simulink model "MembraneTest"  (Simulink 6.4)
settings: Solver=ode45  StartTime=0.0  StopTime=SimTime  FixedStep=1E-2  RelTol=1e-5
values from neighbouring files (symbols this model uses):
  b = S/Sm    (= 0.1)    [Constantes.m]    (also in ConstantesBck.m)
  C = 1    [Constantes.m]    (also in ConstantesBck.m)
  Cmem = 1E-6*Sm*(1-b)    (= 2.826e-08)    [Constantes.m]    (also in ConstantesBck.m = 3.14e-11; ImpedanceZtissus.m = 4e-08; Ztissus.m = 4e-08; CalculCharge.m = 1)
  Fact = 10^2    (= 100)    [Constantes.m]    (also in ConstantesBck.m)
  gk = 36    [Constantes.m]    (also in ConstantesBck.m; sim_hh.m)
  gl = 0.3    [Constantes.m]    (also in ConstantesBck.m; sim_hh.m)
  gna = 120    [Constantes.m]    (also in ConstantesBck.m; sim_hh.m)
  h0 = cdep(4)    [temps.m]    (also in Constantes.m = 0.5961; ConstantesBck.m = 0.5961)
  I0Stim = AddI    (= 0)    [WaveComp.m]    (also in WaveCompIET.m; WaveCompIETAnim.m; WaveCompIETIf.m; WaveCompIETSeul.m = Hm(i)*1E-6)
  m0 = cdep(5)    [temps.m]    (also in Constantes.m = 0.0529; ConstantesBck.m = 0.0529)
  mK = 0    [Constantes.m]    (also in ConstantesBck.m)
  mL = 0    [Constantes.m]    (also in ConstantesBck.m)
  mNa = 0    [Constantes.m]    (also in ConstantesBck.m)
  n0 = 0.3177    [Constantes.m]    (also in ConstantesBck.m)
  Rcan = 6.398E3*Sm*(1-b)    (= 180.80748)    [Constantes.m]    (also in ConstantesBck.m = 0.03454; ImpedanceZtissus.m = 44; Ztissus.m = 44)
  Sm = 3.14e-2    (= 0.0314)    [Constantes.m]    (also in ConstantesBck.m = 0.000314)
  T0Stim = i    [WaveComp.m]    (also in WaveCompIET.m; WaveCompIETAnim.m = 5; WaveCompIETIf.m; WaveCompIETSeul.m = T0Hm(i)*1E-3)
  TypeStim = 5    [WaveComp.m]    (also in WaveCompIET.m; WaveCompIETAnim.m; WaveCompIETIf.m; WaveCompIETSeul.m)
  Vk = -82    [Constantes.m]    (also in ConstantesBck.m)
  Vl = -59    [Constantes.m]    (also in ConstantesBck.m)
  Vna = 45    [Constantes.m]    (also in ConstantesBck.m)
  Vr = -70    [Constantes.m]    (also in ConstantesBck.m)
libraries: simulink x1

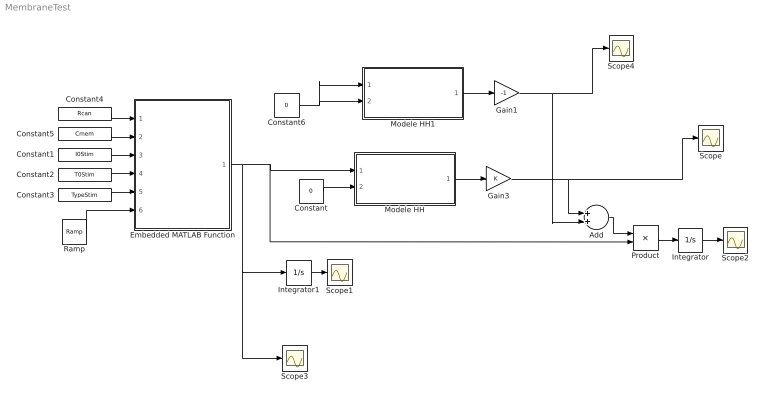
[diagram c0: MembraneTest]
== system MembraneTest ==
  Add : Sum  OutScaling=2^-10
  Constant : Constant  Value=0  OutDataType=sfix(16)  ConRadixGroup=Use specified scaling  OutScaling=2^0  SampleTime=inf  FramePeriod=inf
  Constant1 : Constant  Value=I0Stim  OutDataType=sfix(16)  ConRadixGroup=Use specified scaling  OutScaling=2^0  SampleTime=inf  FramePeriod=inf
  Constant2 : Constant  Value=T0Stim  OutDataType=sfix(16)  ConRadixGroup=Use specified scaling  OutScaling=2^0  SampleTime=inf  FramePeriod=inf
  Constant3 : Constant  Value=TypeStim  OutDataType=sfix(16)  ConRadixGroup=Use specified scaling  OutScaling=2^0  SampleTime=inf  FramePeriod=inf
  Constant4 : Constant  Value=Rcan  OutDataType=sfix(16)  ConRadixGroup=Use specified scaling  OutScaling=2^0  SampleTime=inf  FramePeriod=inf
  Constant5 : Constant  Value=Cmem  OutDataType=sfix(16)  ConRadixGroup=Use specified scaling  OutScaling=2^0  SampleTime=inf  FramePeriod=inf
  Constant6 : Constant  Value=0  OutDataType=sfix(16)  ConRadixGroup=Use specified scaling  OutScaling=2^0  SampleTime=inf  FramePeriod=inf
  Embedded MATLAB Function : Stateflow chart
  Gain1 : Gain  Gain=-1
  Gain3 : Gain
  Integrator : Integrator
  Integrator1 : Integrator
  Modele HH : Subsystem
  Modele HH1 : Subsystem
  Product : Product
  Ramp : simulink/Sources/Ramp  SystemSampleTime=-1  slope=1  start=0  X0=0
  Scope{,1..4} (5 alike) : Scope
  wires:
  Modele HH/1(HHout) -> Gain3/1
  Constant/1 -> Modele HH/2(VRefIn)
  Gain3/1 -> Scope/1, Add/1
  Product/1 -> Integrator/1
  Integrator/1 -> Scope2/1
  Constant1/1 -> Embedded MATLAB Function/3(I0Stim)
  Constant2/1 -> Embedded MATLAB Function/4(T0Stim)
  Constant3/1 -> Embedded MATLAB Function/5(TypeStim)
  Integrator1/1 -> Scope1/1
  Ramp/1 -> Embedded MATLAB Function/6(temps)
  Embedded MATLAB Function/1(Istim) -> Scope3/1, Integrator1/1, Modele HH/1(HHin), Product/2
  Constant4/1 -> Embedded MATLAB Function/1(Rcan)
  Constant5/1 -> Embedded MATLAB Function/2(Cmem)
  Modele HH1/1(HHout) -> Gain1/1
  Constant6/1 -> Modele HH1/2(VRefIn), Modele HH1/1(HHin)
  Gain1/1 -> Add/2, Scope4/1
  Add/1 -> Product/1

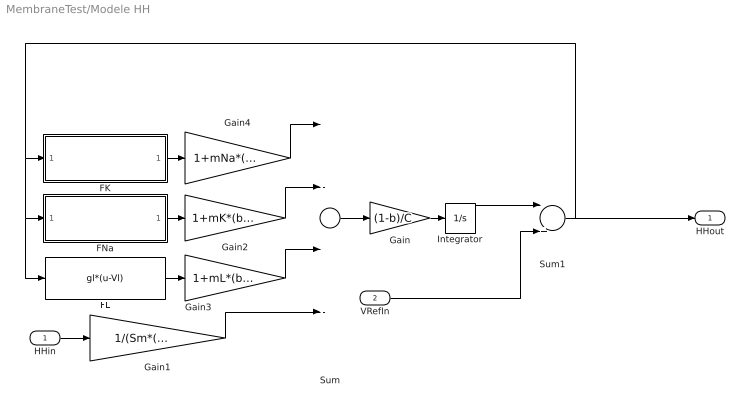
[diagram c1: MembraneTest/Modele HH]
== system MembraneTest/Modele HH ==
  HHin : Inport
  VRefIn : Inport  Port=2
  FK : Subsystem
  FL : Fcn  Expr=gl*(u-Vl)
  FNa : Subsystem
  Gain : Gain  Gain=(1-b)/C
  Gain1 : Gain  Gain=1/(Sm*(1-b)*Fact)
  Gain2 : Gain  Gain=1+mK*(b/(1-b))
  Gain3 : Gain  Gain=1+mL*(b/(1-b))
  Gain4 : Gain  Gain=1+mNa*(b/(1-b))
  Integrator : Integrator  InitialCondition=Vr
  Sum : Sum  Inputs=|---+
  Sum1 : Sum  Inputs=|++
  HHout : Outport
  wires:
  Sum/1 -> Gain/1
  Gain/1 -> Integrator/1
  FK/1(FKout) -> Gain4/1
  FNa/1(FNaOut) -> Gain2/1
  FL/1 -> Gain3/1
  HHin/1 -> Gain1/1
  Integrator/1 -> Sum1/1
  Sum1/1 -> FNa/1(FNaIn), FL/1, FK/1(FKIn), HHout/1
  Gain1/1 -> Sum/4
  Gain4/1 -> Sum/1
  Gain2/1 -> Sum/2
  Gain3/1 -> Sum/3
  VRefIn/1 -> Sum1/2

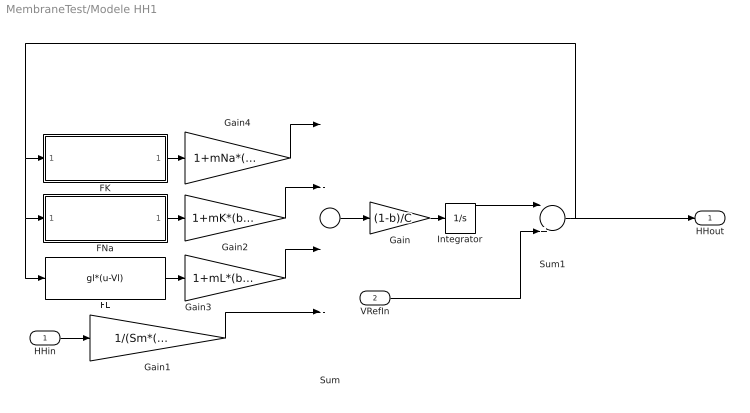
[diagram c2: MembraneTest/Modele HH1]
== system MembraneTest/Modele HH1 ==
  HHin : Inport
  VRefIn : Inport  Port=2
  FK : Subsystem
  FL : Fcn  Expr=gl*(u-Vl)
  FNa : Subsystem
  Gain : Gain  Gain=(1-b)/C
  Gain1 : Gain  Gain=1/(Sm*(1-b)*Fact)
  Gain2 : Gain  Gain=1+mK*(b/(1-b))
  Gain3 : Gain  Gain=1+mL*(b/(1-b))
  Gain4 : Gain  Gain=1+mNa*(b/(1-b))
  Integrator : Integrator  InitialCondition=Vr
  Sum : Sum  Inputs=|---+
  Sum1 : Sum  Inputs=|++
  HHout : Outport
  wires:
  Sum/1 -> Gain/1
  Gain/1 -> Integrator/1
  FK/1(FKout) -> Gain4/1
  FNa/1(FNaOut) -> Gain2/1
  FL/1 -> Gain3/1
  HHin/1 -> Gain1/1
  Integrator/1 -> Sum1/1
  Sum1/1 -> FNa/1(FNaIn), FL/1, FK/1(FKIn), HHout/1
  Gain1/1 -> Sum/4
  Gain4/1 -> Sum/1
  Gain2/1 -> Sum/2
  Gain3/1 -> Sum/3
  VRefIn/1 -> Sum1/2

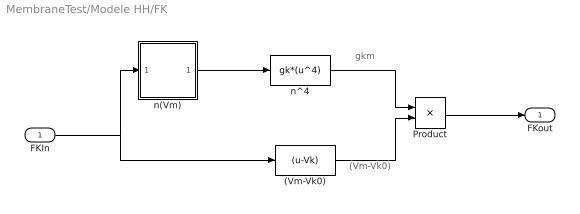
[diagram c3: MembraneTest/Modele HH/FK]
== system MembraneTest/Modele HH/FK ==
  note: gkm
  note: (Vm-Vk0)
  FKIn : Inport
  (Vm-Vk0) : Fcn  Expr=(u-Vk)
  Product : Product
  n(Vm) : Subsystem
  n^4 : Fcn  Expr=gk*(u^4)
  FKout : Outport  InitialOutput=0
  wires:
  n(Vm)/1(n) -> n^4/1
  (Vm-Vk0)/1 -> Product/2
  Product/1 -> FKout/1
  n^4/1 -> Product/1
  FKIn/1 -> n(Vm)/1(Vm), (Vm-Vk0)/1

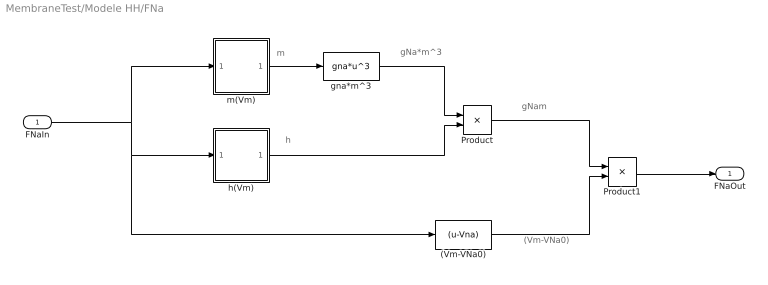
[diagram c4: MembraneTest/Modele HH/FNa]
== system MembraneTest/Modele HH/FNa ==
  note: gNa*m^3
  note: m
  note: h
  note: gNam
  note: (Vm-VNa0)
  FNaIn : Inport
  (Vm-VNa0) : Fcn  Expr=(u-Vna)
  Product : Product
  Product1 : Product
  gna*m^3 : Fcn  Expr=gna*u^3
  h(Vm) : Subsystem
  m(Vm) : Subsystem
  FNaOut : Outport  InitialOutput=0
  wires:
  (Vm-VNa0)/1 -> Product1/2
  gna*m^3/1 -> Product/1
  Product1/1 -> FNaOut/1
  FNaIn/1 -> m(Vm)/1(Vm), h(Vm)/1(Vm), (Vm-VNa0)/1
  m(Vm)/1(n) -> gna*m^3/1
  h(Vm)/1(h) -> Product/2
  Product/1 -> Product1/1

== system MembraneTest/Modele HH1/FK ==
  note: gkm
  note: (Vm-Vk0)
  FKIn : Inport
  (Vm-Vk0) : Fcn  Expr=(u-Vk)
  Product : Product
  n(Vm) : Subsystem
  n^4 : Fcn  Expr=gk*(u^4)
  FKout : Outport  InitialOutput=0
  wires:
  n(Vm)/1(n) -> n^4/1
  (Vm-Vk0)/1 -> Product/2
  Product/1 -> FKout/1
  n^4/1 -> Product/1
  FKIn/1 -> n(Vm)/1(Vm), (Vm-Vk0)/1

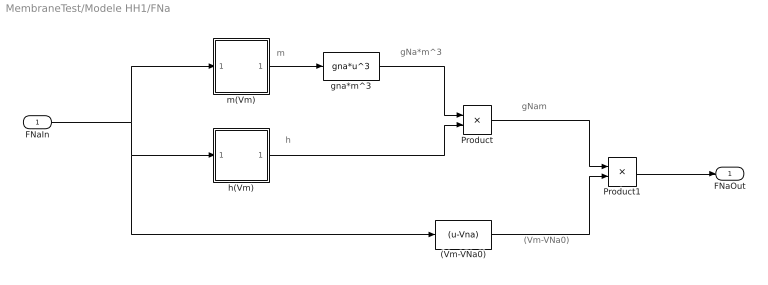
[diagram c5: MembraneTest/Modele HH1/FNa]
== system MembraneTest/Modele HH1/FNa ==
  note: gNa*m^3
  note: m
  note: h
  note: gNam
  note: (Vm-VNa0)
  FNaIn : Inport
  (Vm-VNa0) : Fcn  Expr=(u-Vna)
  Product : Product
  Product1 : Product
  gna*m^3 : Fcn  Expr=gna*u^3
  h(Vm) : Subsystem
  m(Vm) : Subsystem
  FNaOut : Outport  InitialOutput=0
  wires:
  (Vm-VNa0)/1 -> Product1/2
  gna*m^3/1 -> Product/1
  Product1/1 -> FNaOut/1
  FNaIn/1 -> m(Vm)/1(Vm), h(Vm)/1(Vm), (Vm-VNa0)/1
  m(Vm)/1(n) -> gna*m^3/1
  h(Vm)/1(h) -> Product/2
  Product/1 -> Product1/1

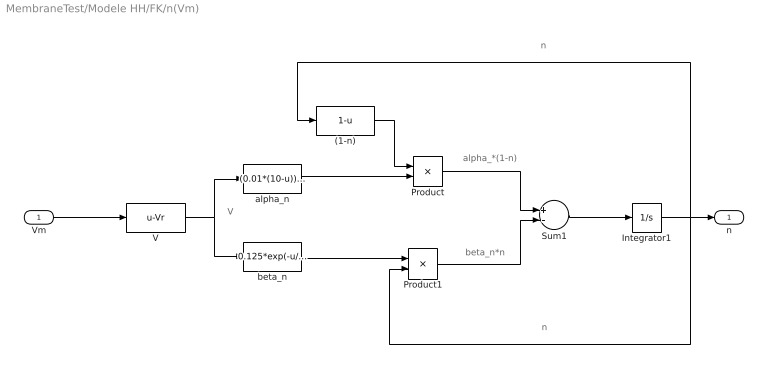
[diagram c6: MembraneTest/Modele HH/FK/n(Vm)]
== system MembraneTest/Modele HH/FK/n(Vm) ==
  note: V
  note: alpha_*(1-n)
  note: beta_n*n
  note: n
  note: n
  Vm : Inport
  (1-n) : Fcn  Expr=1-u
  Integrator1 : Integrator  InitialCondition=n0
  Product : Product
  Product1 : Product
  Sum1 : Sum  Inputs=+-
  V : Fcn  Expr=u-Vr
  alpha_n : Fcn  Expr=(0.01*(10-u))/(exp((10-u)/10)-1)
  beta_n : Fcn  Expr=0.125*exp(-u/80)
  n : Outport  InitialOutput=0
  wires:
  V/1 -> alpha_n/1, beta_n/1
  alpha_n/1 -> Product/2
  (1-n)/1 -> Product/1
  beta_n/1 -> Product1/1
  Product/1 -> Sum1/1
  Product1/1 -> Sum1/2
  Sum1/1 -> Integrator1/1
  Integrator1/1 -> (1-n)/1, Product1/2, n/1
  Vm/1 -> V/1

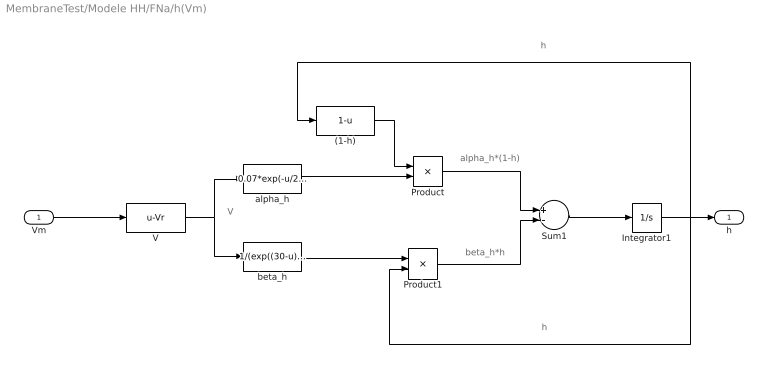
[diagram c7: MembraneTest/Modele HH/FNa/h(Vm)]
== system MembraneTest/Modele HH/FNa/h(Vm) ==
  note: h
  note: h
  note: beta_h*h
  note: alpha_h*(1-h)
  note: V
  Vm : Inport
  (1-h) : Fcn  Expr=1-u
  Integrator1 : Integrator  InitialCondition=h0
  Product : Product
  Product1 : Product
  Sum1 : Sum  Inputs=+-
  V : Fcn  Expr=u-Vr
  alpha_h : Fcn  Expr=0.07*exp(-u/20)
  beta_h : Fcn  Expr=1/(exp((30-u)/10)+1)
  h : Outport  InitialOutput=0
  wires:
  Vm/1 -> V/1
  Integrator1/1 -> h/1, Product1/2, (1-h)/1
  Sum1/1 -> Integrator1/1
  Product1/1 -> Sum1/2
  Product/1 -> Sum1/1
  beta_h/1 -> Product1/1
  (1-h)/1 -> Product/1
  alpha_h/1 -> Product/2
  V/1 -> beta_h/1, alpha_h/1

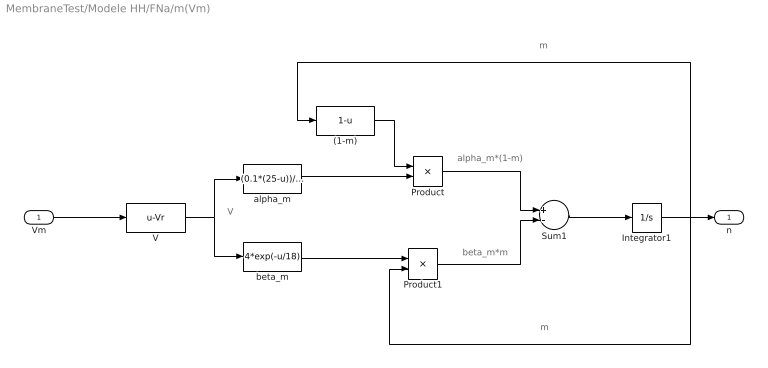
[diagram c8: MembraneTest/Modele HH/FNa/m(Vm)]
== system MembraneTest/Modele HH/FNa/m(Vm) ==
  note: m
  note: m
  note: beta_m*m
  note: alpha_m*(1-m)
  note: V
  Vm : Inport
  (1-m) : Fcn  Expr=1-u
  Integrator1 : Integrator  InitialCondition=m0
  Product : Product
  Product1 : Product
  Sum1 : Sum  Inputs=+-
  V : Fcn  Expr=u-Vr
  alpha_m : Fcn  Expr=(0.1*(25-u))/(exp((25-u)/10)-1)
  beta_m : Fcn  Expr=4*exp(-u/18)
  n : Outport  InitialOutput=0
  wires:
  Vm/1 -> V/1
  Integrator1/1 -> n/1, Product1/2, (1-m)/1
  Sum1/1 -> Integrator1/1
  Product1/1 -> Sum1/2
  Product/1 -> Sum1/1
  beta_m/1 -> Product1/1
  (1-m)/1 -> Product/1
  alpha_m/1 -> Product/2
  V/1 -> beta_m/1, alpha_m/1

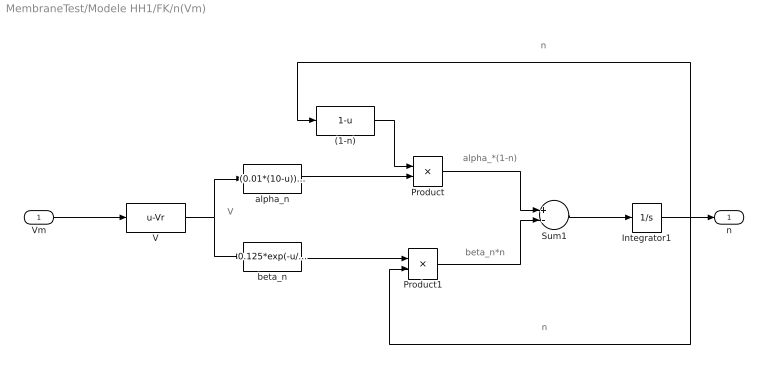
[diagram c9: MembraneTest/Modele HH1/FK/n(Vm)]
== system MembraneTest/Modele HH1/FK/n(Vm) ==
  note: V
  note: alpha_*(1-n)
  note: beta_n*n
  note: n
  note: n
  Vm : Inport
  (1-n) : Fcn  Expr=1-u
  Integrator1 : Integrator  InitialCondition=n0
  Product : Product
  Product1 : Product
  Sum1 : Sum  Inputs=+-
  V : Fcn  Expr=u-Vr
  alpha_n : Fcn  Expr=(0.01*(10-u))/(exp((10-u)/10)-1)
  beta_n : Fcn  Expr=0.125*exp(-u/80)
  n : Outport  InitialOutput=0
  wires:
  V/1 -> alpha_n/1, beta_n/1
  alpha_n/1 -> Product/2
  (1-n)/1 -> Product/1
  beta_n/1 -> Product1/1
  Product/1 -> Sum1/1
  Product1/1 -> Sum1/2
  Sum1/1 -> Integrator1/1
  Integrator1/1 -> (1-n)/1, Product1/2, n/1
  Vm/1 -> V/1

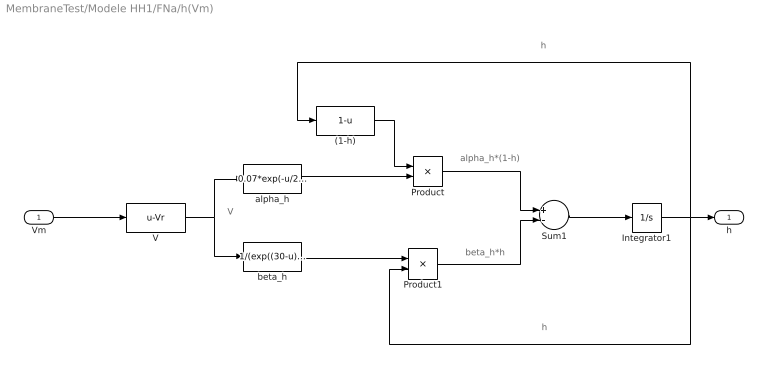
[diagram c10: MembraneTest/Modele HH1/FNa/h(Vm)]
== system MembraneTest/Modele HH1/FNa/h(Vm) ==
  note: h
  note: h
  note: beta_h*h
  note: alpha_h*(1-h)
  note: V
  Vm : Inport
  (1-h) : Fcn  Expr=1-u
  Integrator1 : Integrator  InitialCondition=h0
  Product : Product
  Product1 : Product
  Sum1 : Sum  Inputs=+-
  V : Fcn  Expr=u-Vr
  alpha_h : Fcn  Expr=0.07*exp(-u/20)
  beta_h : Fcn  Expr=1/(exp((30-u)/10)+1)
  h : Outport  InitialOutput=0
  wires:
  Vm/1 -> V/1
  Integrator1/1 -> h/1, Product1/2, (1-h)/1
  Sum1/1 -> Integrator1/1
  Product1/1 -> Sum1/2
  Product/1 -> Sum1/1
  beta_h/1 -> Product1/1
  (1-h)/1 -> Product/1
  alpha_h/1 -> Product/2
  V/1 -> beta_h/1, alpha_h/1

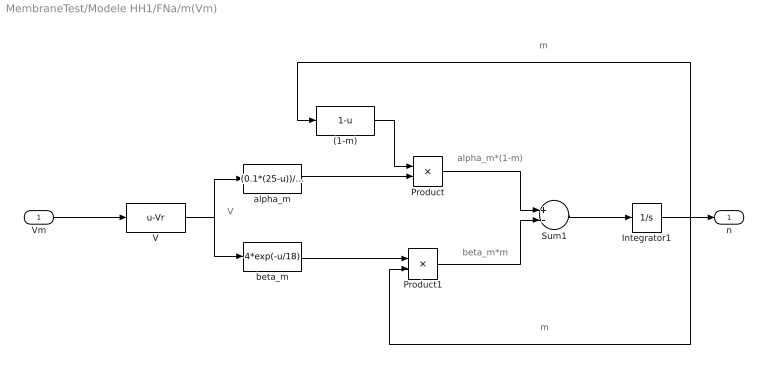
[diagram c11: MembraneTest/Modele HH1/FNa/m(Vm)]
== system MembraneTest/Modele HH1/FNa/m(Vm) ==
  note: m
  note: m
  note: beta_m*m
  note: alpha_m*(1-m)
  note: V
  Vm : Inport
  (1-m) : Fcn  Expr=1-u
  Integrator1 : Integrator  InitialCondition=m0
  Product : Product
  Product1 : Product
  Sum1 : Sum  Inputs=+-
  V : Fcn  Expr=u-Vr
  alpha_m : Fcn  Expr=(0.1*(25-u))/(exp((25-u)/10)-1)
  beta_m : Fcn  Expr=4*exp(-u/18)
  n : Outport  InitialOutput=0
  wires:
  Vm/1 -> V/1
  Integrator1/1 -> n/1, Product1/2, (1-m)/1
  Sum1/1 -> Integrator1/1
  Product1/1 -> Sum1/2
  Product/1 -> Sum1/1
  beta_m/1 -> Product1/1
  (1-m)/1 -> Product/1
  alpha_m/1 -> Product/2
  V/1 -> beta_m/1, alpha_m/1

== matlab function Embedded
MATLAB Function ==
function Istim = courant(Rcan,Cmem,I0Stim,T0Stim,TypeStim,temps)
% This block supports an embeddable subset of the MATLAB language.
% See the help menu for details. 
taum = 1/(30.4E-3)*1E-6*1000;
if temps <= T0Stim
    if TypeStim == 0
        Iout = I0Stim;
    elseif TypeStim == 1
        Iout = I0Stim*exp(temps/taum);
    elseif TypeStim == 2
        Iout = I0Stim*sin(pi/T0Stim*temps);
    elseif TypeStim == 3
        Iout = I0Stim*sin(pi/(2*T0Stim)*temps);
    elseif TypeStim == 4
        Iout = I0Stim*sinh(temps/taum);
    else
        Iout = I0Stim*(sin(pi/T0Stim*temps)+1/3*sin(3*pi/T0Stim*temps));
    end
else
    Iout = 0;
end
Istim = Iout;
